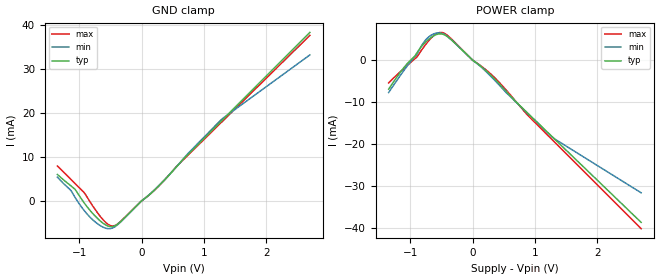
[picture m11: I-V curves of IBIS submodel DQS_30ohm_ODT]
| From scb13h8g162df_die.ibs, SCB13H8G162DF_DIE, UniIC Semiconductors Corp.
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|   Submodel DQS_30ohm_ODT
[Submodel] DQS_30ohm_ODT
Submodel_type Dynamic_clamp
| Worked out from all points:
|   GND clamp passes 1 mA (typ) near -0.07 V on its own axis
|   POWER clamp passes 1 mA (typ) near -0.07 V on its own axis
[GND_clamp]
|Voltage   I(typ)   I(min)   I(max)
-1.35V    6.012mA    5.397mA    7.93mA
-1.125V   3.311mA    2.207mA    4.775mA
-1.069V   2.659mA    843.4uA    3.973mA
-928mV    -313uA     -2.062mA   2mA
-759mV    -3.247mA   -4.611mA   -1.655mA
-563mV    -5.583mA   -6.271mA   -5.068mA
-478mV    -5.883mA   -6.245mA   -5.714mA
-422mV    -5.654mA   -5.851mA   -5.588mA
253mV     3.09mA     3.124mA    3.054mA
562mV     7.774mA    7.825mA    7.854mA
1.294V    18.39mA    18.69mA    18.06mA
2.7V      38.37mA    33.24mA    37.7mA
[POWER_clamp]
|Voltage   I(typ)   I(min)   I(max)
-1.35V    -6.858mA   -7.656mA   -5.385mA
-1.125V   -2.099mA   -2.821mA   -2.201mA
-900mV    1.715mA    1.365mA    744.6uA
-816mV    3.421mA    3.649mA    2.567mA
-731mV    4.71mA     5.25mA     4.247mA
-591mV    6.093mA    6.465mA    6.255mA
-450mV    6.041mA    6.112mA    6.392mA
100nV     -189.5nA   -185.3nA   -197.4nA
338mV     -4.272mA   -4.54mA    -3.942mA
872mV     -12.45mA   -12.51mA   -12.93mA
1.294V    -18.48mA   -18.51mA   -19.19mA
2.7V      -38.56mA   -31.52mA   -40.06mA
